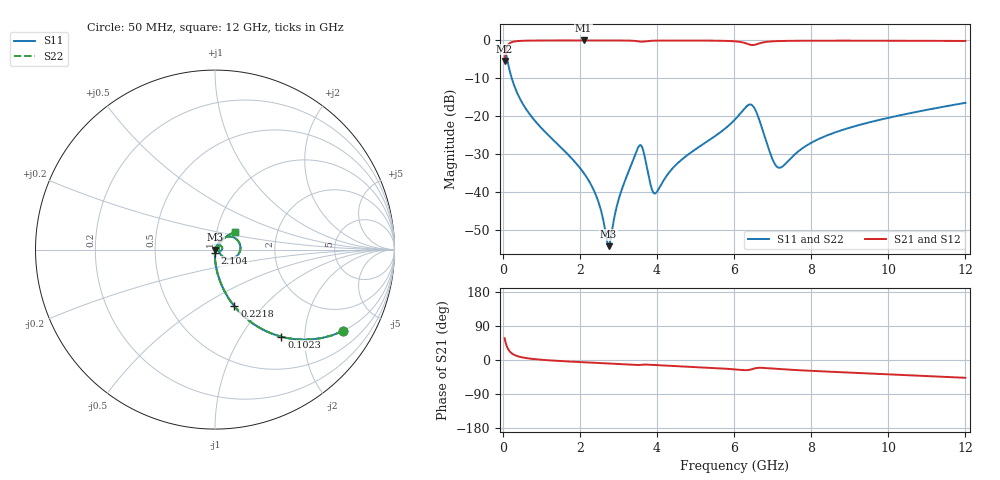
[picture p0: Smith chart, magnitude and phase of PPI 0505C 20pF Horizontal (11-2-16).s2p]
# MHz S MA R 50
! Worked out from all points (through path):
!   1601 points, 50 MHz to 12 GHz, reference 50 ohm
!   highest |S21| = -0.01 dB at 2.096 GHz (marker M1); lowest = -5.4 dB at 50 MHz (marker M2)
!   group delay of S21, straight-line fit = 12.3 ps
!   lowest |S11| = -54.3 dB at 2.746 GHz (marker M3), VSWR 1.00, Z = 50.2 - j0.0471 ohm
!   |S11| at or under -10 dB: 235.4 MHz to end of sweep
!   |S22| runs from -54.3 to -1.5 dB; largest |S21 - S12| = 0
!   S11 on the Smith chart (normalised r, x): 50 MHz: 0.99, -3.14; 102.3 MHz: 0.99, -1.54; 221.8 MHz: 0.99, -0.71; 2.104 GHz: 1.00, -0.04; 12 GHz: 1.23, +0.25
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50  0.8448 -32.5  0.535 57.5  0.535 57.5  0.8448 -32.5
102.2812  0.6106 -52.7  0.7916 37.3  0.7916 37.3  0.6106 -52.7
221.7812  0.3337 -71.2  0.9422 18.8  0.9422 18.8  0.3337 -71.2
707.25  0.1048 -85.9  0.9936 3.7  0.9936 3.7  0.1048 -85.9
2044.156  0.01947 -91.7  0.9983 -5.7  0.9983 -5.7  0.01947 -91.7
2096.438  0.01792 -91.5  0.9983 -5.9  0.9983 -5.9  0.01792 -91.5
2103.906  0.0177 -91.5  0.9983 -6.0  0.9983 -6.0  0.0177 -91.5
2462.406  0.007903 -86.1  0.9982 -7.7  0.9982 -7.7  0.007903 -86.1
2746.219  0.001918 -14.2  0.9979 -9.1  0.9979 -9.1  0.001918 -14.2
3052.438  0.009451 61.5  0.9969 -10.6  0.9969 -10.6  0.009451 61.5
3537.906  0.04043 26.2  0.9682 -13.2  0.9682 -13.2  0.04043 26.2
3642.469  0.0355 -7.8  0.9644 -12.2  0.9644 -12.2  0.0355 -7.8
3888.938  0.0102 0.6  0.9898 -13.0  0.9898 -13.0  0.0102 0.6
4038.312  0.01073 39.6  0.9933 -13.9  0.9933 -13.9  0.01073 39.6
4561.125  0.0245 64.3  0.9955 -16.5  0.9955 -16.5  0.0245 64.3
6025  0.09035 50.3  0.9725 -24.8  0.9725 -24.8  0.09035 50.3
6488.062  0.1365 -7.5  0.8676 -23.5  0.8676 -23.5  0.1365 -7.5
6995.938  0.02713 -28.0  0.9725 -22.8  0.9725 -22.8  0.02713 -28.0
7152.781  0.02088 0.6  0.9805 -23.9  0.9805 -23.9  0.02088 0.6
8019.156  0.04496 51.6  0.991 -28.7  0.991 -28.7  0.04496 51.6
10013.31  0.09528 49.2  0.9898 -37.8  0.9898 -37.8  0.09528 49.2
12000  0.1498 41.1  0.983 -47.0  0.983 -47.0  0.1498 41.1
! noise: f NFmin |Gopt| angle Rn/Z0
50  0.0003884  0.8658  1.119  0.0006218
1372  0.003921  0.6697  4.776  0.002278
2701  0.007151  0.6488  8.976  0.003843
4031  0.0162  0.7549  13.32  0.01317
5360  0.01748  0.7078  17.5  0.0115
6682  0.07355  0.9042  21.93  0.1623
8012  0.02454  0.6963  25.97  0.01501
9341  0.02222  0.6285  29.79  0.01051
1.067e+04  0.02301  0.6017  33.51  0.009822
1.2e+04  0.02465  0.5903  37.13  0.009971
